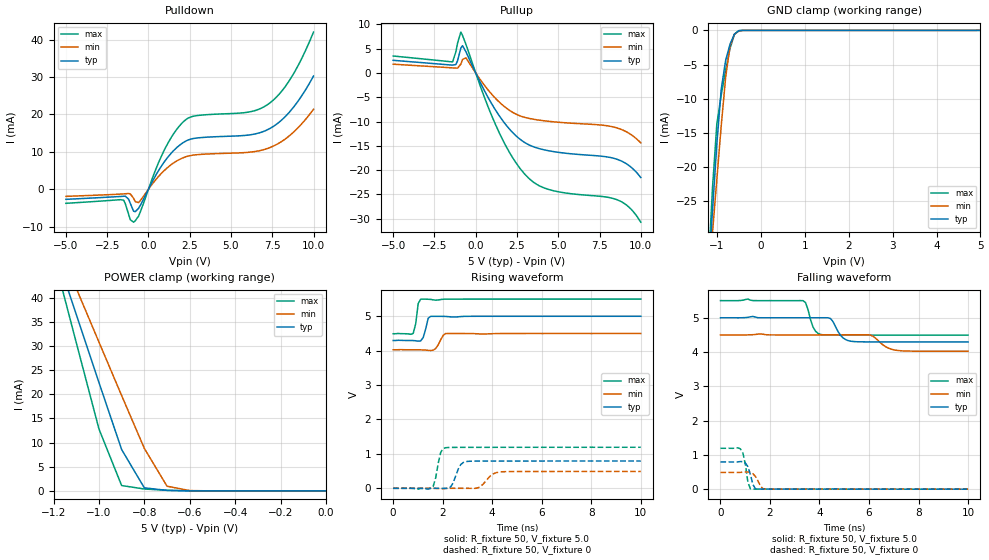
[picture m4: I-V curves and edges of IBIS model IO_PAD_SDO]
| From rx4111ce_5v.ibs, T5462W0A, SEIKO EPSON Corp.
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[Model]   IO_PAD_SDO
Model_type 3-state
Enable Active-High
Polarity Non-Inverting
Vmeas=2.5
C_comp   2.5p   2.0p   3.0p
[Temperature Range] 25   105   -40
[Voltage Range]   5.0   4.5   5.5
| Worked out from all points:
|   slope of the pulldown table from 0 to 0.75 V, typ, clamps not added: 126 ohm
|   slope of the pullup table from 0 to 0.75 V, typ, clamps not added: 149 ohm
|   GND clamp passes 1 mA (typ) near -0.63 V on its own axis
|   POWER clamp passes 1 mA (typ) near -0.80 V on its own axis
|   falling waveform, R_fixture 50, V_fixture 5.0: 20-80 % time 356ps typ, 506ps min, 262ps max; typ from 5 V to 4.29 V
|   falling waveform, R_fixture 50, V_fixture 0: 20-80 % time 184ps typ, 226ps min, 165ps max; typ from 0.793 V to 0 V
|   rising waveform, R_fixture 50, V_fixture 5.0: 20-80 % time 153ps typ, 215ps min, 120ps max; typ from 4.29 V to 5 V
|   rising waveform, R_fixture 50, V_fixture 0: 20-80 % time 264ps typ, 390ps min, 201ps max; typ from 0 V to 0.793 V
[Pullup]
-5V       2.598mA    1.8mA      3.487mA
-1.4V     1.602mA    1.04mA     2.29mA
-1.2V     1.734mA    995.1uA    4.356mA
-900mV    5.146mA    1.814mA    8.407mA
-600mV    4.408mA    3.126mA    5.954mA
1.2V      -7.642mA   -5.236mA   -10.62mA
2.1V      -11.76mA   -7.82mA    -16.67mA
3V        -14.38mA   -9.175mA   -20.93mA
4.5V      -16.07mA   -9.985mA   -24.05mA
8.6V      -17.81mA   -11.36mA   -26.14mA
9.4V      -19.36mA   -12.67mA   -27.99mA
10V       -21.52mA   -14.39mA   -30.71mA
[Pulldown]
-5V       -2.695mA   -1.898mA   -3.76mA
-1.5V     -1.871mA   -1.232mA   -2.909mA
-1.1V     -3.756mA   -1.223mA   -8.144mA
-900mV    -5.868mA   -2.416mA   -8.805mA
-600mV    -5.116mA   -3.564mA   -7.202mA
900mV     6.952mA    4.772mA    9.936mA
2V        12.16mA    8.239mA    17.55mA
2.7V      13.56mA    9.131mA    19.52mA
6.1V      14.52mA    9.905mA    20.68mA
7.3V      16.12mA    11.05mA    22.91mA
8.6V      20.94mA    14.54mA    29.51mA
10V       30.29mA    21.41mA    42.04mA
[GND Clamp]
-5V       -428.8mA   -348.1mA   -527.7mA
-1.2V     -36.43mA   -37.5mA    -35.6mA
-1.1V     -26.48mA   -29.64mA   -23.15mA
-1V       -16.59mA   -21.78mA   -13.65mA
-900mV    -8.58mA    -13.93mA   -9.45mA
-800mV    -4.393mA   -6.884mA   -5.813mA
-700mV    -2.03mA    -2.311mA   -2.637mA
-600mV    -545.2uA   -558.8uA   -605.7uA
-500mV    -56.87uA   -90.58uA   -35.51uA
-300mV    -121.9nA   -876.6nA   -9.379nA
5V        101.4pA    6.061uA    84.58pA
[POWER Clamp]
-5V       593.9mA    482.2mA    740.2mA
-1.2V     50.66mA    53.08mA    48.75mA
-1.1V     36.55mA    41.95mA    30.73mA
-1V       22.47mA    30.83mA    12.85mA
-900mV    8.574mA    19.75mA    1.117mA
-800mV    640.7uA    8.813mA    397uA
-700mV    110.3uA    975.9uA    130.4uA
-600mV    21.48uA    71.72uA    21uA
0V        101.4pA    787.2pA    98.23pA
[Falling Waveform]
R_fixture=50
V_fixture=5.0
V_fixture_min=4.5
V_fixture_max=5.5
0s        5V         4.5V       5.5V
3.333ns   5V         4.5V       5.499V
3.737ns   5V         4.5V       4.732V
4.141ns   5V         4.5V       4.502V
4.444ns   4.977V     4.5V       4.494V
4.848ns   4.49V      4.5V       4.493V
5.253ns   4.317V     4.5V       4.493V
6.061ns   4.297V     4.493V     4.493V
7.172ns   4.296V     4.044V     4.492V
10ns      4.295V     4.024V     4.492V
[Falling Waveform]
R_fixture=50
V_fixture=0
V_fixture_min=0
V_fixture_max=0
0s        793.4mV    489.5mV    1.193V
808.1ps   805.9mV    490.4mV    1.175V
909.1ps   801.4mV    495.1mV    1.049V
1.01ns    759.1mV    499.4mV    708mV
1.111ns   654.4mV    500mV      191.8mV
1.212ns   421.8mV    487.3mV    9.92mV
1.414ns   10.78mV    371.8mV    3.229mV
1.616ns   2.303mV    96.01mV    2.932mV
1.818ns   1.944mV    4.715mV    2.696mV
10ns      93.16uV    87.95uV    92.16uV
[Rising Waveform]
R_fixture=50
V_fixture=5.0
V_fixture_min=4.5
V_fixture_max=5.5
0s        4.295V     4.024V     4.492V
808.1ps   4.294V     4.025V     4.5V
909.1ps   4.288V     4.024V     4.781V
1.01ns    4.277V     4.024V     5.369V
1.111ns   4.283V     4.023V     5.497V
1.212ns   4.382V     4.021V     5.497V
1.414ns   4.944V     4.01V      5.495V
1.515ns   4.998V     4.005V     5.49V
2.121ns   4.995V     4.498V     5.498V
10ns      5V         4.5V       5.5V
[Rising Waveform]
R_fixture=50
V_fixture=0
V_fixture_min=0
V_fixture_max=0
0s        0V         0V         0V
1.515ns   -648.3uV   9.036uV    66.86uV
1.717ns   100uV      -3.66mV    305.9mV
1.919ns   -848.3uV   -11.49mV   1.045V
2.121ns   -2.503mV   -2.97mV    1.18V
2.323ns   41.81mV    -10.17uV   1.187V
2.929ns   775.3mV    -782.4uV   1.19V
3.434ns   790.3mV    17.4mV     1.191V
4.343ns   792mV      477.2mV    1.191V
10ns      793.2mV    489.3mV    1.193V
[Ramp]
R_load=50
dV/dt_r   4.759E-1/2.547E-10   2.936E-1/3.737E-10   7.156E-1/1.803E-10
dV/dt_f   4.227E-1/3.486E-10   2.855E-1/5.054E-10   6.048E-1/2.464E-10
|[End   IO_PAD_SDO
